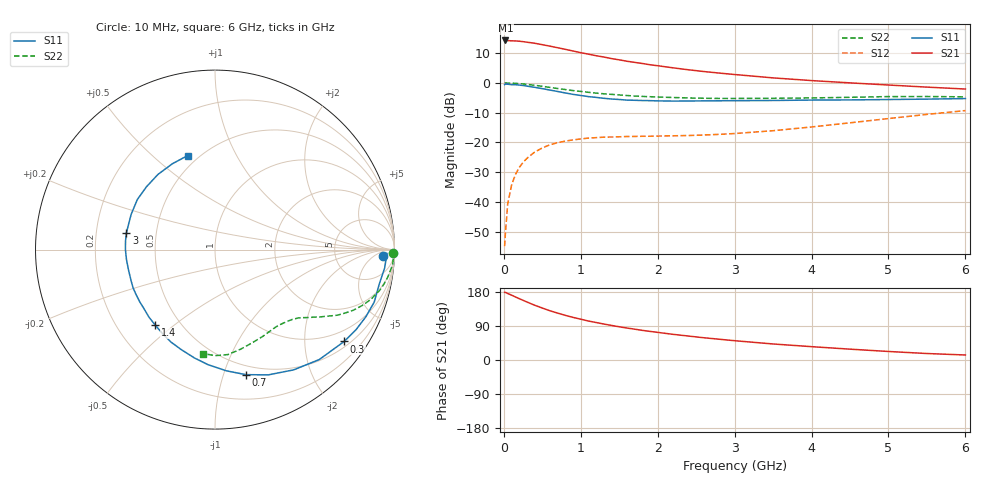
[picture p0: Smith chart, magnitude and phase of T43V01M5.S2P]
! Infineon Technologies  Discrete & RF Semiconductors
! BFR182T
! Si NPN RF Bipolar Junction Transistor in SC75
! VCE = 3 V  IC = 1.5 mA
! Common Emitter S-Parameters:  October  1999
# GHz  S  MA  R  50
!  f  S11  S21  S12  S22
! GHz  MAG  ANG  MAG  ANG  MAG  ANG  MAG  ANG
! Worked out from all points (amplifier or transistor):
!   36 points, 10 MHz to 6 GHz, reference 50 ohm
!   highest |S21| = 14.3 dB at 20 MHz (marker M1)
!   |S21| within 3 dB of that: start of sweep to 802.7 MHz
!   unconditionally stable (mu >= 1): 2.166 GHz to 4.437 GHz
!   at 250 MHz: K = 0.11, MSG = 20.3 dB, |S12| = -26.7 dB
!   at 1.4 GHz: K = 0.69, MSG = 13.2 dB, |S12| = -18.2 dB
!   at 6 GHz: K = 0.83, MSG = 3.6 dB, |S12| = -9.3 dB
!   S11 on the Smith chart (normalised r, x): 10 MHz: 23, -13; 300 MHz: 0.65, -3.01; 700 MHz: 0.41, -1.19; 1.4 GHz: 0.36, -0.43; 3 GHz: 0.33, +0.08; 6 GHz: 0.44, +0.65
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0.01  0.9366 -2.2  5.114 178.5  0.0018 84.7  0.991 -1.2
0.02  0.9582 -1.2  5.175 178.5  0.0029 91.7  0.9999 -1.0
0.05  0.9509 -6.1  5.148 175.5  0.0092 90.0  0.9955 -2.5
0.1  0.9353 -11.7  5.103 171.2  0.019 83.7  0.9929 -4.8
0.2  0.9203 -23.9  5.026 161.9  0.0378 77.2  0.9726 -9.5
0.3  0.8832 -35.4  4.839 153.1  0.0539 70.4  0.9467 -13.7
0.4  0.8443 -46.5  4.644 144.6  0.0687 64.1  0.9119 -17.7
0.5  0.8007 -56.8  4.393 137.1  0.0807 59.2  0.8773 -20.8
0.6  0.7584 -67.0  4.149 129.9  0.0914 54.8  0.841 -23.7
0.7  0.7173 -76.2  3.903 123.7  0.0989 51.3  0.8049 -26.1
0.9  0.6421 -93.5  3.44 112.4  0.1101 44.8  0.743 -29.8
1.1  0.5884 -108.5  3.046 102.8  0.1183 40.7  0.6951 -32.7
1.4  0.5367 -128.3  2.566 91.2  0.1232 37.0  0.6422 -36.1
1.6  0.5144 -140.4  2.316 84.3  0.1256 36.2  0.6142 -38.1
1.8  0.5059 -150.7  2.121 78.2  0.1268 36.1  0.5931 -40.3
2.2  0.4951 -166.8  1.793 67.7  0.1291 37.9  0.5687 -44.5
2.6  0.4991 180.0  1.554 58.7  0.1331 41.7  0.5523 -49.4
3  0.5024 169.2  1.385 50.9  0.141 46.3  0.5479 -54.2
3.5  0.5068 157.2  1.215 42.3  0.1572 52.0  0.5519 -61.2
4.5  0.5179 137.5  1.002 28.6  0.2134 58.6  0.573 -75.6
5.5  0.534 116.4  0.85 17.1  0.2956 58.0  0.5908 -89.9
6  0.5456 106.2  0.789 13.2  0.3427 55.2  0.583 -96.5
